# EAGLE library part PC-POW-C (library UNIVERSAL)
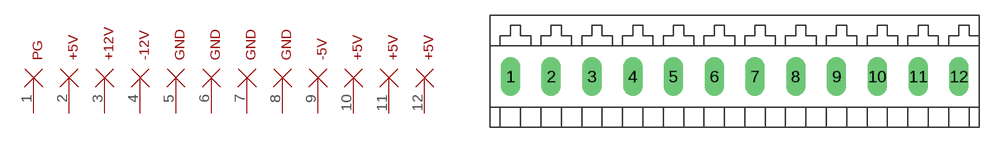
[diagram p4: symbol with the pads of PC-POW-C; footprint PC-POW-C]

Designator prefix CON

## PC-POW-C  [PC-POW-C]
1  P$1
2  P$2
3  P$3
4  P$4
5  P$5
6  P$6
7  P$7
8  P$8
9  P$9
10  P$10
11  P$11
12  P$12

## Footprint PC-POW-C (pad centres in mm)
drill 0.813 pad 1.905 long: 1 0,0; 2 4,0; 3 8,0; 4 12,0; 5 16,0; 6 20,0; 7 24,0; 8 28,0; 9 32,0; 10 36,0; 11 40,0; 12 44,0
